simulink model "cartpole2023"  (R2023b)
settings: Solver=VariableStepAuto  StartTime=0.0  StopTime=20  RelTol=1e-3
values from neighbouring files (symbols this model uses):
  A = [0,1,0,0 ; 0,-d1, -g*m/M,0 ; 0,0,0,1 ; 0,d1/L,q_,-d2]    [cartpole_main.m]    (also in cp_kalman.m; time_varying_LQR.m = [0,1,0,0 ; 0,-d1,f_23, f_24; 0,0,0,1; 0, f_42, f_43, f_44 ]; cp_kalman_extended.m = [0,1,0,0 ; 0,-d1,f_23, f_24; 0,0,0,1; 0, f_42, f_43, f_44 ])
  B = [0, 1.0/M, 0., -1/(M*L)].'    [cartpole_main.m]    (also in cp_kalman.m; time_varying_LQR.m = [0; cp_kalman_extended.m = [0)
  C = [C_cart; C_angle]    [cartpole_main.m]
  P_k_init = .01    (= 0.01)    [cartpole_main.m]
  q1 = 5e-4    (= 0.0005)    [cartpole_main.m]
  q2 = 1e-3    (= 0.001)    [cartpole_main.m]
  Q_ctrl = diag([10,5,20,10])    [cartpole_main.m]
  r1 = 1e-3    (= 0.001)    [cartpole_main.m]
  r2 = 5e-4    (= 0.0005)    [cartpole_main.m]
  R_ctrl = 10    [cartpole_main.m]
  Ts = 0.01    [cartpole_main.m]    (also in cp_kalman.m = in(4); time_varying_LQR.m = in(11); cp_kalman_extended.m = in(4))
  x0 = [0,0,0.5, .1]    [cartpole_main.m]
undefined symbols (not defined in the file or in its folder): K_lqr
libraries: simulink x2

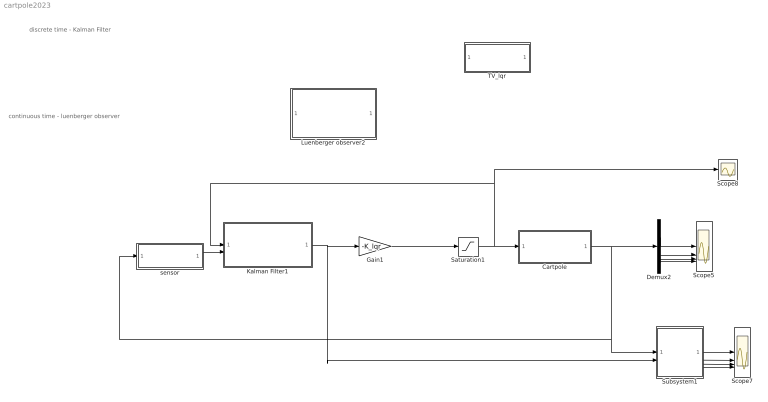
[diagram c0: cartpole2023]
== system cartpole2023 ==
  note: continuous time - luenberger observer
  note: discrete time - Kalman Filter
  Cartpole : Subsystem
  Demux2 : Demux
  Gain1 : Gain  Gain=-K_lqr  Multiplication=Matrix(K*u)
  Kalman Filter1 : Subsystem  TreatAsAtomicUnit=on  SystemSampleTime=Ts
  Luenberger observer2 : Subsystem  Commented=on
  Saturation1 : Saturate  UpperLimit=10  LowerLimit=-10
  Scope5 : Scope  NumInputPorts=4
  Scope7 : Scope  NumInputPorts=4
  Scope8 : Scope
  Subsystem1 : Subsystem
  TV_lqr : Subsystem  Commented=on  TreatAsAtomicUnit=on
  sensor : Subsystem
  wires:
  Subsystem1/1(x1) -> Scope7/1
  Subsystem1/3(x3) -> Scope7/3
  Subsystem1/4(x4) -> Scope7/4
  Subsystem1/2(x2) -> Scope7/2
  Cartpole/1(x) -> Demux2/1, Subsystem1/1(x), sensor/1(x)
  Demux2/4 -> Scope5/4
  Demux2/3 -> Scope5/3
  Demux2/2 -> Scope5/2
  Demux2/1 -> Scope5/1
  Saturation1/1 -> Cartpole/1(u), Scope8/1, Kalman Filter1/1(u)
  Kalman Filter1/1(x_est) -> Gain1/1, Subsystem1/2(x_hat)
  sensor/1(y) -> Kalman Filter1/2(y)
  Gain1/1 -> Saturation1/1

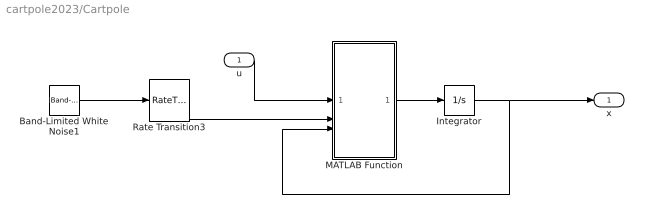
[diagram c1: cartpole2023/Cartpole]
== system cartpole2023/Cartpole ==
  u : Inport
  Band-Limited White Noise1 : simulink/Sources/Band-Limited White Noise  Cov=[q1,q2]  Ts=Ts  seed=[23341]
  Integrator : Integrator  InitialCondition=x0
  MATLAB Function : MATLAB Function  TreatAsAtomicUnit=on
  Rate Transition3 : RateTransition
  x : Outport
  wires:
  MATLAB Function/1(y) -> Integrator/1
  Integrator/1 -> MATLAB Function/3(s), x/1
  u/1 -> MATLAB Function/1(u)
  Rate Transition3/1 -> MATLAB Function/2(n)
  Band-Limited White Noise1/1 -> Rate Transition3/1

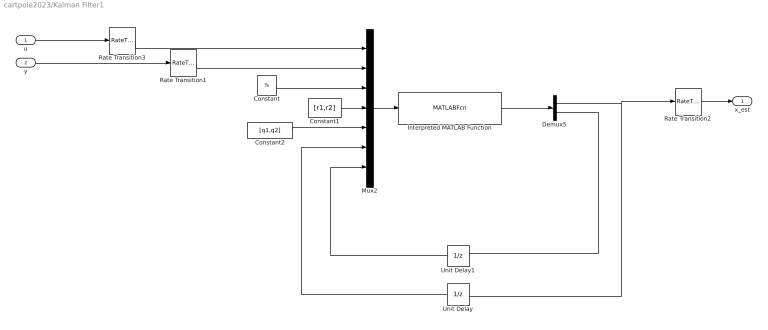
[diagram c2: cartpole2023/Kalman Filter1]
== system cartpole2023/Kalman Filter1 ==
  u : Inport
  y : Inport  Port=2
  Constant : Constant  Value=Ts
  Constant1 : Constant  Value=[r1,r2]
  Constant2 : Constant  Value=[q1,q2]
  Demux5 : Demux  Outputs=[4, 16]
  Interpreted MATLAB Function : MATLABFcn  MATLABFcn=cp_kalman_extended  OutputDimensions=20
  Mux2 : Mux  Inputs=7
  Rate Transition1 : RateTransition  OutPortSampleTime=Ts
  Rate Transition2 : RateTransition
  Rate Transition3 : RateTransition  OutPortSampleTime=Ts
  Unit Delay : UnitDelay  InitialCondition=x0  SampleTime=-1  HasFrameUpgradeWarning=on
  Unit Delay1 : UnitDelay  InitialCondition=reshape( P_k_init*eye(4),[16,1])  SampleTime=-1  HasFrameUpgradeWarning=on
  x_est : Outport
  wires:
  Unit Delay1/1 -> Mux2/7
  Demux5/1 -> Rate Transition2/1, Unit Delay/1
  y/1 -> Rate Transition1/1
  Demux5/2 -> Unit Delay1/1
  Interpreted MATLAB Function/1 -> Demux5/1
  u/1 -> Rate Transition3/1
  Unit Delay/1 -> Mux2/6
  Mux2/1 -> Interpreted MATLAB Function/1
  Constant/1 -> Mux2/3
  Constant1/1 -> Mux2/4
  Constant2/1 -> Mux2/5
  Rate Transition3/1 -> Mux2/1
  Rate Transition1/1 -> Mux2/2
  Rate Transition2/1 -> x_est/1

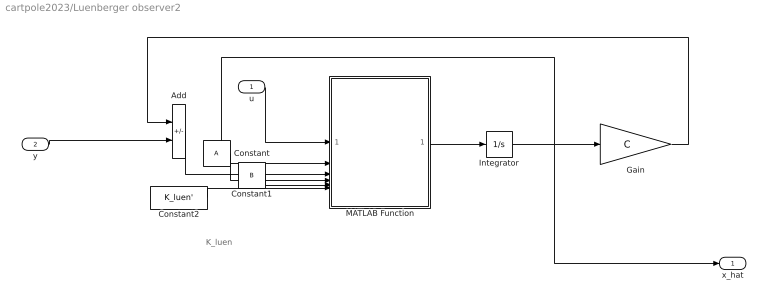
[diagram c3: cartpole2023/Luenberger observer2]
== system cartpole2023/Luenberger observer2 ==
  note: K_luen
  u : Inport
  y : Inport  Port=2
  Add : Sum  Inputs=-+
  Constant : Constant  Value=A
  Constant1 : Constant  Value=B
  Constant2 : Constant  Value=K_luen'
  Gain : Gain  Gain=C  Multiplication=Matrix(K*u)
  Integrator : Integrator  InitialCondition=[0,0,0,0]
  MATLAB Function : MATLAB Function  TreatAsAtomicUnit=on
  x_hat : Outport
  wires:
  Constant/1 -> MATLAB Function/4(A)
  Constant1/1 -> MATLAB Function/5(B)
  Constant2/1 -> MATLAB Function/6(L)
  MATLAB Function/1(x_dot) -> Integrator/1
  Integrator/1 -> MATLAB Function/2(x), Gain/1, x_hat/1
  Gain/1 -> Add/1
  Add/1 -> MATLAB Function/3(e)
  u/1 -> MATLAB Function/1(u)
  y/1 -> Add/2

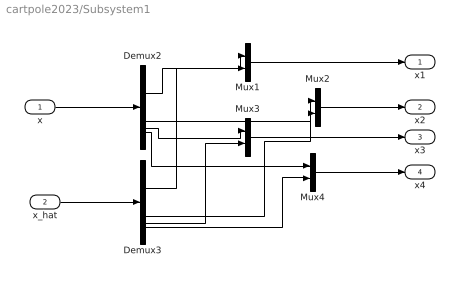
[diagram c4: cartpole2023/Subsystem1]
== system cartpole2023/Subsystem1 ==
  x : Inport
  x_hat : Inport  Port=2
  Demux2 : Demux
  Demux3 : Demux
  Mux{1..4} (4 alike) : Mux  Inputs=2
  x1 : Outport
  x2 : Outport  Port=2
  x3 : Outport  Port=3
  x4 : Outport  Port=4
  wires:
  Demux2/3 -> Mux3/1
  Demux3/4 -> Mux4/2
  x/1 -> Demux2/1
  Mux2/1 -> x2/1
  Demux2/1 -> Mux1/1
  x_hat/1 -> Demux3/1
  Demux3/2 -> Mux2/2
  Demux2/4 -> Mux4/1
  Demux3/3 -> Mux3/2
  Demux2/2 -> Mux2/1
  Mux3/1 -> x3/1
  Demux3/1 -> Mux1/2
  Mux4/1 -> x4/1
  Mux1/1 -> x1/1

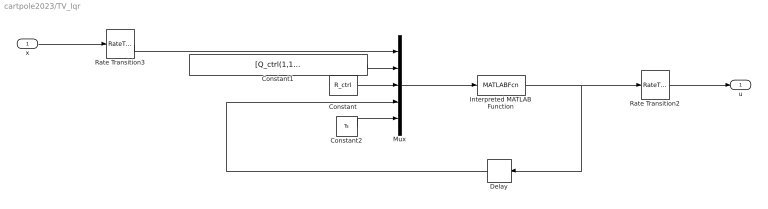
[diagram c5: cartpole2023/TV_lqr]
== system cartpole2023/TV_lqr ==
  x : Inport
  Constant : Constant  Value=R_ctrl
  Constant1 : Constant  Value=[Q_ctrl(1,1),Q_ctrl(2,2),Q_ctrl(3,3),Q_ctrl(4,4)]
  Constant2 : Constant  Value=Ts
  Delay : Delay  DelayLength=1  InitialCondition=0
  Interpreted MATLAB Function : MATLABFcn  MATLABFcn=time_varying_LQR
  Mux : Mux  Inputs=5
  Rate Transition2 : RateTransition
  Rate Transition3 : RateTransition  OutPortSampleTime=Ts
  u : Outport
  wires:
  Interpreted MATLAB Function/1 -> Delay/1, Rate Transition2/1
  x/1 -> Rate Transition3/1
  Mux/1 -> Interpreted MATLAB Function/1
  Constant/1 -> Mux/3
  Constant1/1 -> Mux/2
  Delay/1 -> Mux/4
  Rate Transition3/1 -> Mux/1
  Rate Transition2/1 -> u/1
  Constant2/1 -> Mux/5

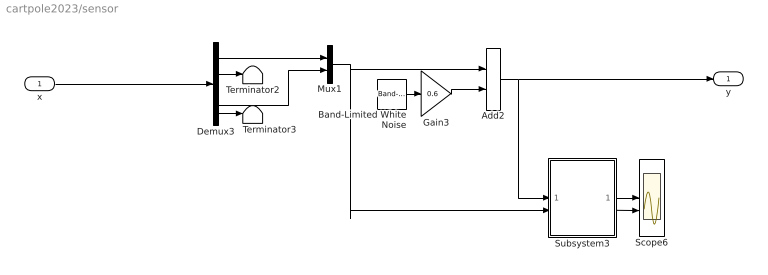
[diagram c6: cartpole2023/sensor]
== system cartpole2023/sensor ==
  x : Inport
  Add2 : Sum
  Band-Limited White Noise : simulink/Sources/Band-Limited White Noise  Cov=[r1,r2]  Ts=Ts  seed=[8451]
  Demux3 : Demux
  Gain3 : Gain  Gain=0.6
  Mux1 : Mux  Inputs=2
  Scope6 : Scope  NumInputPorts=2
  Subsystem3 : Subsystem
  Terminator2 : Terminator
  Terminator3 : Terminator
  y : Outport
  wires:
  Demux3/4 -> Terminator3/1
  Demux3/2 -> Terminator2/1
  Demux3/3 -> Mux1/2
  Add2/1 -> y/1, Subsystem3/1(y_noise)
  Subsystem3/2(y2) -> Scope6/2
  x/1 -> Demux3/1
  Gain3/1 -> Add2/2
  Mux1/1 -> Subsystem3/2(y), Add2/1
  Subsystem3/1(y1) -> Scope6/1
  Demux3/1 -> Mux1/1
  Band-Limited White Noise/1 -> Gain3/1

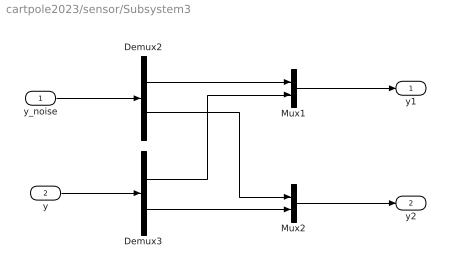
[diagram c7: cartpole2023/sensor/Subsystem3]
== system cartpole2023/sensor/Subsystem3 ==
  y_noise : Inport
  y : Inport  Port=2
  Demux2 : Demux  Outputs=2
  Demux3 : Demux  Outputs=2
  Mux1 : Mux  Inputs=2
  Mux2 : Mux  Inputs=2
  y1 : Outport
  y2 : Outport  Port=2
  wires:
  Mux1/1 -> y1/1
  Demux3/1 -> Mux1/2
  Demux2/2 -> Mux2/1
  Demux3/2 -> Mux2/2
  y/1 -> Demux3/1
  Demux2/1 -> Mux1/1
  Mux2/1 -> y2/1
  y_noise/1 -> Demux2/1

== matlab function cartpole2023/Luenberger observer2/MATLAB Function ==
function x_dot = fcn(u,x,e,A,B,L)

x_dot = A*x + B*u + L*e;

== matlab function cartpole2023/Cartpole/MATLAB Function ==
function y = fcn(u,n,s)

dot_x = s(2) ;
theta = s(3) ;
dot_theta = s(4) ;

m = 0.1;
L = 1;
g = 9.81;
M = 1;
d1 = 1;
d2 = 0.5;


x_ddot = u  + m*L*dot_theta^2 * sin(theta) - m*g*cos(theta) *  sin(theta) ;
x_ddot = x_ddot / ( M+m-m* cos(theta)^2 )  + n(1) - d1*dot_x;

theta_ddot = (g*sin( theta ) -  cos( theta )*x_ddot ) / L  + n(2) - d2*dot_theta ;


y = [ dot_x, x_ddot , dot_theta, theta_ddot  ];
